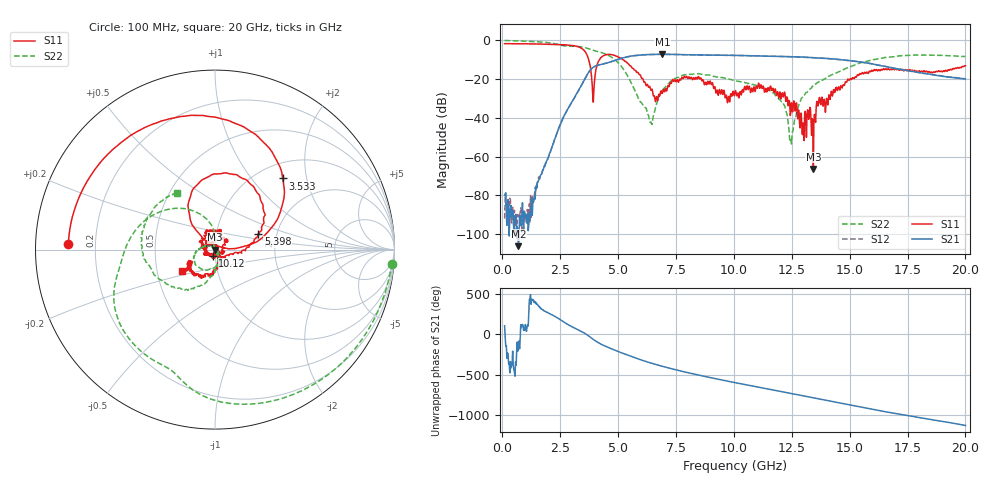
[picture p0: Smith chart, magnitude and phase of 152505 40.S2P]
!  2-Port S-parameters saved by WinCal
! VAR MeasName=S-Parameters (CALIBRATED_DATA) read from VNA (N5230C)
! VAR MeasDate=4/10/2015 9:32:27 AM
! VAR NAME=152505 40
! VAR FILENAME=152505 40.S2P
! VAR DATE=4/10/2015 9:32:27 AM
! VAR PHYS_PORTS=1,2
# Hz S DB R 50
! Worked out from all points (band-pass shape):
!   801 points, 100 MHz to 20 GHz, reference 50 ohm
!   highest |S21| = -7.21 dB at 6.916 GHz (marker M1); lowest = -106.1 dB at 697 MHz (marker M2)
!   |S21| within 3 dB of the highest: 4.897 GHz to 14.78 GHz (9.886 GHz wide, 100 % of centre)
!   lowest |S11| = -66.4 dB at 13.43 GHz (marker M3), VSWR 1.00, Z = 50 + j0.0388 ohm
!   |S11| at or under -10 dB: 3.731 GHz to 4.195 GHz (464 MHz wide, 11.7 % of centre); 5.207 GHz to end of sweep
!   |S22| runs from -53.5 to -0.1 dB; largest |S21 - S12| = 0.0048
!   S11 on the Smith chart (normalised r, x): 100 MHz: 0.10, +0.02; 3.533 GHz: 1.29, +1.46; 5.398 GHz: 1.60, +0.30; 10.12 GHz: 0.97, -0.07; 20 GHz: 0.67, -0.17
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1e8  -1.75 177.6  -80.01 104.1  -91.94 -16.6  -0.09 -4.5
6.97e8  -1.80 163.4  -106.12 -175.0  -91.37 108.1  -0.33 -28.3
1.3935e9  -1.89 146.1  -80.67 44.3  -79.11 40.6  -0.67 -56.6
3.43325e9  -4.21 57.4  -22.84 31.4  -22.83 31.7  -3.44 -141.7
3.53275e9  -5.23 46.4  -20.57 15.5  -20.58 15.5  -3.67 -147.3
3.93075e9  -31.90 95.9  -13.89 -64.7  -13.87 -64.6  -5.21 -167.8
4.353625e9  -8.04 100.1  -12.23 -135.9  -12.24 -136.2  -6.61 169.6
5.398375e9  -11.80 19.8  -8.52 102.7  -8.52 102.6  -18.08 96.4
6.393375e9  -24.74 -44.1  -7.32 5.8  -7.33 5.8  -42.24 58.8
6.741625e9  -28.58 -138.2  -7.24 -23.3  -7.23 -23.5  -30.00 -46.3
6.91575e9  -27.34 -160.9  -7.21 -37.0  -7.24 -37.1  -25.91 -60.5
8.681875e9  -20.50 70.3  -7.56 -157.7  -7.58 -157.9  -17.68 -152.2
1.005e10  -26.56 -111.6  -7.78 121.4  -7.79 121.4  -20.77 179.0
1.012462e10  -28.63 -110.0  -7.80 117.2  -7.81 117.4  -21.08 177.1
1.179125e10  -25.06 136.1  -8.25 25.2  -8.25 24.9  -28.34 148.1
1.246288e10  -36.89 59.7  -8.45 -11.9  -8.52 -12.0  -50.97 -126.4
1.288575e10  -37.70 47.9  -8.63 -34.9  -8.65 -35.0  -30.94 -66.3
1.338325e10  -40.42 -27.3  -8.94 -62.7  -8.91 -62.5  -23.90 -73.7
1.3433e10  -66.39 54.0  -8.96 -65.7  -8.89 -65.4  -23.58 -73.0
1.370662e10  -29.43 -46.2  -9.16 -81.2  -9.21 -81.1  -21.06 -77.3
1.669162e10  -14.80 -131.9  -13.83 114.2  -13.79 113.8  -8.70 -158.9
2e10  -13.13 -146.7  -19.96 -47.5  -19.87 -47.4  -8.41 123.9
